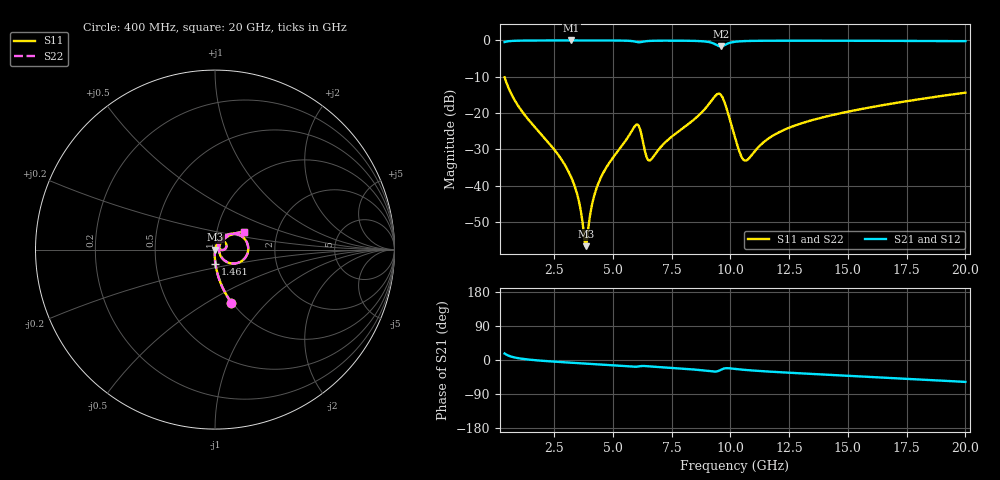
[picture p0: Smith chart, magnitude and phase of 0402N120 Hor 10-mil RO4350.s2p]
# GHz S MA R 50
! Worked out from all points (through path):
!   1960 points, 400 MHz to 20 GHz, reference 50 ohm
!   highest |S21| = -0.01 dB at 3.231 GHz (marker M1); lowest = -1.7 dB at 9.595 GHz (marker M2)
!   group delay of S21, straight-line fit = 8.51 ps
!   lowest |S11| = -56.6 dB at 3.852 GHz (marker M3), VSWR 1.00, Z = 50.1 - j0.0274 ohm
!   |S11| at or under -10 dB: start of sweep to end of sweep
!   |S22| runs from -56.6 to -10.2 dB; largest |S21 - S12| = 0
!   S11 on the Smith chart (normalised r, x): 400 MHz: 0.99, -0.65; 1.461 GHz: 0.99, -0.16; 20 GHz: 1.36, +0.28
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0.4  0.31 -72.8  0.9502 17.1  0.9502 17.1  0.31 -72.8
1.460541  0.07808 -88.4  0.996 0.9  0.996 0.9  0.07808 -88.4
2.641143  0.0278 -92.5  0.9983 -4.9  0.9983 -4.9  0.0278 -92.5
3.231445  0.01316 -91.5  0.9985 -7.1  0.9985 -7.1  0.01316 -91.5
3.491577  0.007555 -87.7  0.9985 -8.1  0.9985 -8.1  0.007555 -87.7
3.671669  0.003947 -77.8  0.9984 -8.8  0.9984 -8.8  0.003947 -77.8
3.851761  0.00148 -10.6  0.9984 -9.4  0.9984 -9.4  0.00148 -10.6
4.151914  0.00617 64.3  0.9982 -10.5  0.9982 -10.5  0.00617 64.3
4.442062  0.01192 69.7  0.9979 -11.5  0.9979 -11.5  0.01192 69.7
5.932823  0.06571 42.9  0.9659 -17.7  0.9659 -17.7  0.06571 42.9
6.132925  0.06377 11.1  0.9428 -16.6  0.9428 -16.6  0.06377 11.1
6.513119  0.0226 20.5  0.9816 -16.6  0.9816 -16.6  0.0226 20.5
6.943338  0.03132 56.4  0.9912 -18.6  0.9912 -18.6  0.03132 56.4
9.134456  0.1389 39.6  0.9417 -29.6  0.9417 -29.6  0.1389 39.6
9.594691  0.1791 -10.6  0.8257 -25.9  0.8257 -25.9  0.1791 -10.6
10.205  0.04567 -47.8  0.9578 -23.6  0.9578 -23.6  0.04567 -47.8
10.46514  0.02558 -25.2  0.974 -25.2  0.974 -25.2  0.02558 -25.2
10.67524  0.02232 5.1  0.9805 -26.4  0.9805 -26.4  0.02232 5.1
11.80582  0.04893 49.3  0.9902 -31.1  0.9902 -31.1  0.04893 49.3
13.46667  0.07983 49.4  0.9909 -36.8  0.9909 -36.8  0.07983 49.4
16.73834  0.133 40.8  0.986 -47.3  0.986 -47.3  0.133 40.8
20  0.1913 30.9  0.9763 -57.8  0.9763 -57.8  0.1913 30.9
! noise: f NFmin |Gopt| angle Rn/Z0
0.4  0.00124  0.7828  1.543  0.001172
2.571  0.004499  0.645  6.451  0.002392
4.752  0.00846  0.6511  11.49  0.004566
6.933  0.01945  0.7648  16.79  0.01645
9.104  0.05293  0.8801  21.97  0.09213
11.29  0.02836  0.7452  27.08  0.02117
13.47  0.02193  0.6361  31.74  0.01055
15.64  0.02182  0.5925  36.22  0.00893
17.82  0.02287  0.5703  40.58  0.008552
20  0.02434  0.5583  44.78  0.008568
